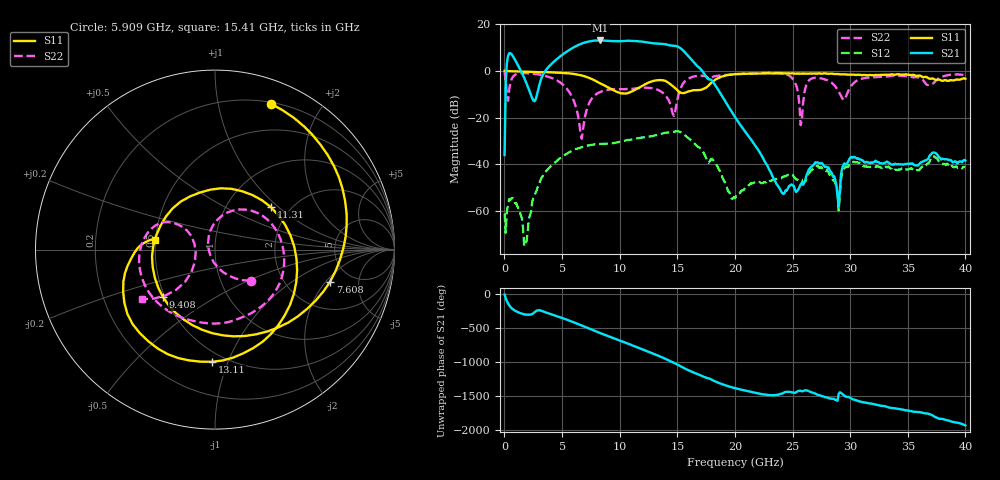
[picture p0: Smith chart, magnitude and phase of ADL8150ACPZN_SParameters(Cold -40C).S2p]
! Analog Devices, Inc.
! Device:	ADL8150ACPZN
! Description:	"GaAs, HBT, MMIC, Low Phase Noise Amplifier, 6 GHz to 14 GHz"
! Conditions:	Vcc = 5.0 V
!		Icc = 74 mA quiescent (Self-biased mode)
!		Pin = -20 dBm
!		Operating Temperature = -40 C (at package bottom)
! Product validation unit SN19 soldered down to Evaluation Board as shown on ADL8150-EVALZ User Guide. Board loss de-embedded from S21 magnitude.  All other RF measurements reference to RF coaxial connector.
! Frequency (GHz)	S11_Mag (dB)	S11_Phase (deg)	S21_Mag (dB)	S21_Phase (deg)	S12_Mag (dB)	S12_Phase (deg)	S22_Mag (dB)	S22_Phase (deg)
#  GHZ  S  DB  R 50
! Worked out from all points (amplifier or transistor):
!   401 points, 10 MHz to 40 GHz, reference 50 ohm
!   highest |S21| = 13.1 dB at 8.308 GHz (marker M1)
!   |S21| within 3 dB of that: 5.991 GHz to 15.17 GHz (9.184 GHz wide, 86.8 % of centre)
!   unconditionally stable (mu >= 1): start of sweep to end of sweep
!   at 6.608 GHz: K = 2.07, MAG = 16.3 dB, |S12| = -32.8 dB
!   at 20 GHz: K = 196.94, MAG = -8.5 dB, |S12| = -54.6 dB
!   at 40 GHz: K = 876.38, MAG = -31.0 dB, |S12| = -41.2 dB
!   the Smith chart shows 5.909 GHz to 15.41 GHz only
!   S11 on the Smith chart (normalised r, x): 5.909 GHz: 0.21, +1.43; 7.608 GHz: 3.47, -2.22; 9.408 GHz: 0.49, -0.30; 11.31 GHz: 1.60, +0.89; 13.11 GHz: 0.43, -0.88; 15.41 GHz: 0.50, +0.06
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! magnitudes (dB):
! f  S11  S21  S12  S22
! 10 MHz  0.0  -36.0  -61.1  -0.2
! 509.9 MHz  -0.1  7.6  -55.3  -5.1
! 1.81 GHz  -0.3  -4.1  -73.9  -1.0
! 3.309 GHz  -0.5  -1.9  -45.1  -1.9
! 5.909 GHz  -1.2  9.9  -34.1  -11.6
! 6.708 GHz  -1.9  11.8  -32.7  -29.0
! 7.608 GHz  -3.5  12.9  -31.6  -11.6
! 8.308 GHz  -5.3  13.1  -31.3  -9.0
! 9.408 GHz  -8.1  12.8  -31.0  -7.8
! 11.31 GHz  -8.1  12.8  -29.1  -7.5
! 13.11 GHz  -4.1  11.8  -27.6  -7.7
! 13.41 GHz  -3.9  11.7  -27.2  -8.3
! 14.71 GHz  -6.9  10.8  -26.0  -19.3
! 15.41 GHz  -9.4  9.2  -26.6  -6.2
! 20.1 GHz  -1.3  -20.5  -53.6  -1.4
! 24.1 GHz  -1.0  -52.3  -45.6  -1.0
! 25.7 GHz  -1.1  -48.6  -46.6  -23.2
! 26.7 GHz  -1.1  -40.8  -42.4  -3.1
! 28.9 GHz  -1.3  -53.2  -52.9  -8.0
! 30.1 GHz  -1.6  -36.8  -39.2  -6.3
! 33.4 GHz  -1.6  -39.5  -41.5  -2.2
! 40 GHz  -3.3  -38.4  -41.2  -1.8
